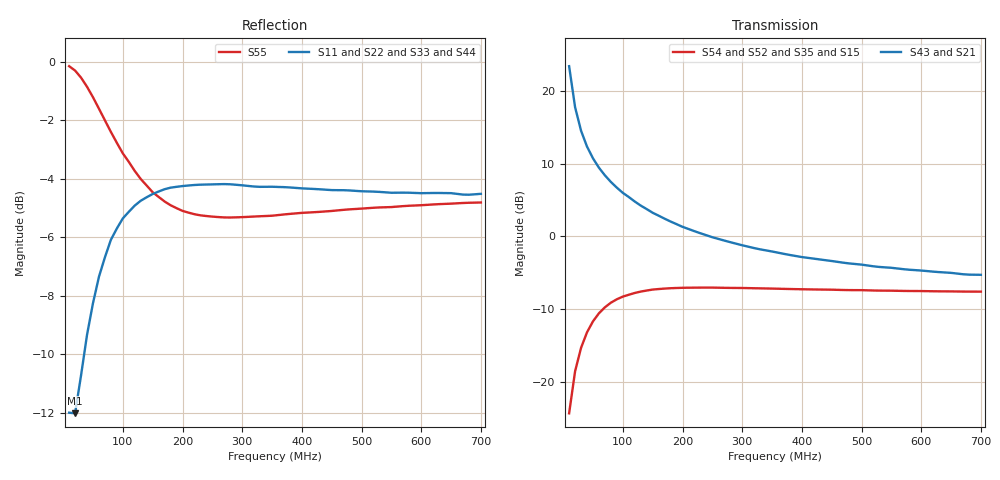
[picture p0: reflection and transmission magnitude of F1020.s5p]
! Date: Mon Aug 07 16:49:04 1995
!  POLYFET RF DEVICES
!  F1020 (Each Side)
!  S PARAMETERS
!  VDS=28V, IDQ=1.00A
!AWR Design Environment (2053) Wed Feb 04 14:30:09 2004
!freq-unit  param-type  data-format  keyword  impedance-ohms
# MHz  S  MA  R  50
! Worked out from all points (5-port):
!   70 points, 10 MHz to 700 MHz, reference 50 ohm
!   strongest paths, dB at 10 MHz, 180 MHz, 360 MHz, 530 MHz, 700 MHz:
!     S43: 23.4, 2.1, -2.2, -4.2, -5.3
!     S21: 23.4, 2.1, -2.2, -4.2, -5.3
!     S54: -24.3, -7.1, -7.2, -7.4, -7.6
!     S52: -24.3, -7.1, -7.2, -7.4, -7.6
!     S35: -24.1, -7.0, -7.1, -7.5, -7.7
!     S15: -24.1, -7.0, -7.1, -7.5, -7.7
!   lowest |S11| = -12.0 dB at 20 MHz (marker M1), VSWR 1.67, Z = 45.7 - j24.4 ohm
!   |S11| at or under -10 dB: start of sweep to 35.19 MHz
